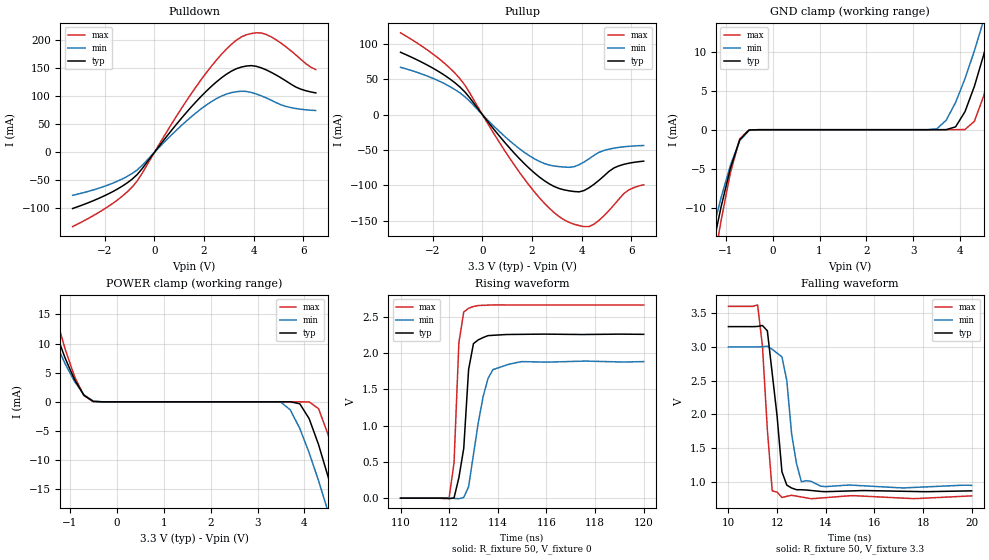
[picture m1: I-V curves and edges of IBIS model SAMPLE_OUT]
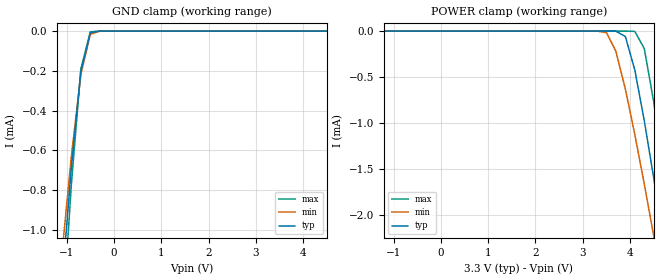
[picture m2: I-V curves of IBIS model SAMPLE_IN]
[IBIS Ver]   4.0
[File Name]   iqsample.ibs
[File Rev]   1.0
[Date]   09/21/2004
[Source]   State secret, can't reveal that.
[Notes]   This IBIS file was created to provide an instructive
   sample for learning to use the IBIS Quality Checklist.
[Copyright]   Unauthorized reproduction and/or distribution is strictly
   prohibited by no one.
[Disclaimer]   This info is for modeling purposes only and is not guaranteed.
   Do not bend, fold, spindle, mutilate, or swallow.
[Component]   IQ_SAMPLE
[Manufacturer]  ACME Inc.
[Package]
|   typ   min   max
R_pkg   0.042   0.034   0.051
L_pkg   2.620nH   2.429nH   2.867nH
C_pkg   0.311pF   0.284pF   0.341pF
[Pin]   signal_name   model_name
1   CLKIN   SAMPLE_IN
2   OE   SAMPLE_OE
3   GND   GND
4   1YP   SAMPLE_OUT
5   1YN   SAMPLE_OUT
6   VDD   POWER
7   1YP   SAMPLE_OUT
8   1YN   SAMPLE_OUT
| Models and submodels in the file (3): SAMPLE_OUT (Output), SAMPLE_IN (Input), SAMPLE_OE (Input)
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[Model]   SAMPLE_OUT
Model_type   Output
Polarity   Non-Inverting
Enable   Active-High
Vmeas = 1.5V
Cref = 5pF
Rref = 500
Vref = 0
|   typ   min   max
C_comp   2.8pF   NA   9pF
[Voltage range]   3.3   3.0   3.6
[Temperature range]   40   0   85
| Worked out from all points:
|   slope of the pulldown table from 0 to 0.495 V, typ, clamps not added: 17.4 ohm
|   slope of the pullup table from 0 to 0.495 V, typ, clamps not added: 22.3 ohm
|   GND clamp passes 1 mA (typ) near -0.65 V on its own axis
|   POWER clamp passes 1 mA (typ) near -0.68 V on its own axis
|   rising waveform, R_fixture 50, V_fixture 0: 20-80 % time 335ps typ, 584ps min, 193ps max; typ from 0 V to 2.26 V
|   falling waveform, R_fixture 50, V_fixture 3.3: 20-80 % time 416ps typ, 410ps min, 303ps max; typ from 3.3 V to 0.867 V
[Pullup]
|   Voltage   I(typ)   I(min)   I(max)
-3.3V     88.24mA    67mA       115.7mA
-1.9V     63.84mA    49.93mA    83.25mA
-900mV    38.85mA    30.58mA    50.64mA
1.7V      -69.67mA   -53.61mA   -91.53mA
2.5V      -93.58mA   -69.21mA   -125.5mA
3.3V      -106.5mA   -74.18mA   -149mA
3.9V      -109.3mA   -70.83mA   -157mA
4.3V      -103.5mA   -62.44mA   -158.4mA
4.7V      -92.88mA   -53.34mA   -149.5mA
5.3V      -75.51mA   -47.45mA   -127.9mA
5.9V      -68.76mA   -44.83mA   -106.6mA
6.5V      -65.87mA   -43.68mA   -99.27mA
[Pulldown]
|   Voltage   I(typ)   I(min)   I(max)
-3.3V     -100.2mA   -76.67mA   -132.4mA
-1.9V     -75.01mA   -58.78mA   -97.6mA
-900mV    -47.82mA   -37.74mA   -61.93mA
1.1V      61.3mA     48.29mA    79.08mA
1.9V      100.5mA    78.08mA    130.6mA
2.7V      132.7mA    100.2mA    174.5mA
3.5V      151.9mA    108.8mA    205.5mA
4.1V      153.2mA    104mA      212.9mA
4.5V      146.9mA    96.98mA    210mA
5.3V      127.1mA    81.76mA    187.9mA
5.9V      112.5mA    76.69mA    165.6mA
6.5V      105.8mA    74.44mA    147.3mA
[GND Clamp]
|   Voltage   I(typ)   I(min)   I(max)
-3.3V     -89.26mA   -75.29mA   -109.5mA
-1.3V     -15.72mA   -13.54mA   -18.89mA
-1.1V     -9.954mA   -8.748mA   -11.72mA
-700mV    -1.28mA    -1.396mA   -1.169mA
-500mV    -41.84uA   -85.02uA   -18.78uA
3.5V      20.1nA     113.8uA    10.65nA
3.9V      365.2uA    3.496mA    61.69nA
4.1V      2.311mA    6.532mA    29.64uA
4.5V      9.621mA    14.08mA    4.347mA
4.7V      14.27mA    18.37mA    9.059mA
4.9V      19.37mA    22.89mA    14.71mA
6.5V      68.27mA    63.5mA     75.98mA
[POWER Clamp]
|   Voltage   I(typ)   I(min)   I(max)
-3.3V     71.55mA    58.24mA    93.72mA
-1.7V     22.04mA    18.36mA    27.9mA
-1.5V     16.77mA    14.08mA    21.05mA
-900mV    3.809mA    3.496mA    4.347mA
-500mV    60.1uA     113.8uA    29.64uA
3.5V      -28.72nA   -85.02uA   -19.28nA
4.1V      -2.893mA   -8.748mA   -18.78uA
4.3V      -7.339mA   -13.54mA   -1.169mA
4.5V      -12.76mA   -18.79mA   -5.544mA
4.7V      -18.82mA   -24.37mA   -11.72mA
4.9V      -25.35mA   -30.24mA   -18.88mA
6.5V      -85.32mA   -81.98mA   -90.15mA
[ramp]
| variable   typ   min   max
dV/dt_r   1.3634E+00/3.2045E-10  1.1382E+00/5.9005E-10  1.6021E+00/1.9338E-10
dV/dt_f   1.4862E+00/4.2439E-10  1.2600E+00/3.7876E-10  1.7300E+00/2.8615E-10
[Rising Waveform]
R_fixture = 50
V_fixture = 0
|   Time   V(typ)   V(min)   V(max)
110ns     0V         0V         -1.462uV
112ns     -7.478mV   1.194mV    10.71mV
112.2ns   2.378mV    -2.799mV   482.2mV
112.4ns   281.9mV    -7.451mV   2.139V
112.6ns   685.4mV    9.597mV    2.563V
112.8ns   1.771V     158.6mV    2.614V
113ns     2.128V     601mV      2.64V
113.4ns   2.212V     1.402V     2.655V
113.8ns   2.242V     1.769V     2.66V
120ns     2.256V     1.88V      2.66V
[Falling Waveform]
R_fixture = 50
V_fixture = 3.3
V_fixture_min = 3.0
V_fixture_max = 3.6
|   Time   V(typ)   V(min)   V(max)
10ns      3.3V       3V         3.6V
11.2ns    3.303V     2.999V     3.622V
11.4ns    3.317V     3.003V     3.008V
11.6ns    3.239V     3.009V     1.775V
11.8ns    2.608V     2.965V     868.1mV
12.2ns    1.151V     2.851V     769.7mV
12.4ns    952.8mV    2.503V     786.9mV
12.6ns    909.4mV    1.706V     802mV
13ns      884.1mV    1.002V     776.7mV
20ns      867.4mV    948.2mV    793.1mV
[Model]   SAMPLE_IN
Model_type   Input
Polarity   Non-Inverting
Vinl = 0.8V
Vinh = 2.0V
|   typ   min   max
C_comp   2.5pF   NA   6pF
[Voltage Range]   3.3   3.0   3.6
[Temperature range]   40   0   85
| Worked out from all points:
|   GND clamp passes 1 mA (typ) near -1.01 V on its own axis
[GND Clamp]
|   Voltage   I(typ)   I(min)   I(max)
-3.3V     -9.387mA   -7.872mA   -11.61mA
-1.1V     -1.278mA   -1.123mA   -1.509mA
-900mV    -684.4uA   -628.5uA   -770.6uA
-700mV    -203.7uA   -218.5uA   -190.1uA
-500mV    -8.062uA   -16.38uA   -3.548uA
-300mV    -36.49nA   -171.5nA   -6.088nA
6.5V      3.916nA    3.963nA    3.913nA
[POWER Clamp]
|   Voltage   I(typ)   I(min)   I(max)
-3.3V     3.976nA    3.842nA    4.154nA
3.3V      0A         -171.5nA   180.7pA
3.5V      -1.679nA   -16.38uA   60.25pA
3.7V      -647.2nA   -218.5uA   -63.24pA
3.9V      -59.34uA   -628.5uA   -6.088nA
4.1V      -422.5uA   -1.123mA   -3.548uA
4.3V      -972.4uA   -1.66mA    -190.1uA
4.5V      -1.596mA   -2.225mA   -770.6uA
4.7V      -2.262mA   -2.809mA   -1.509mA
4.9V      -2.955mA   -3.41mA    -2.317mA
6.5V      -8.993mA   -8.532mA   -9.667mA
